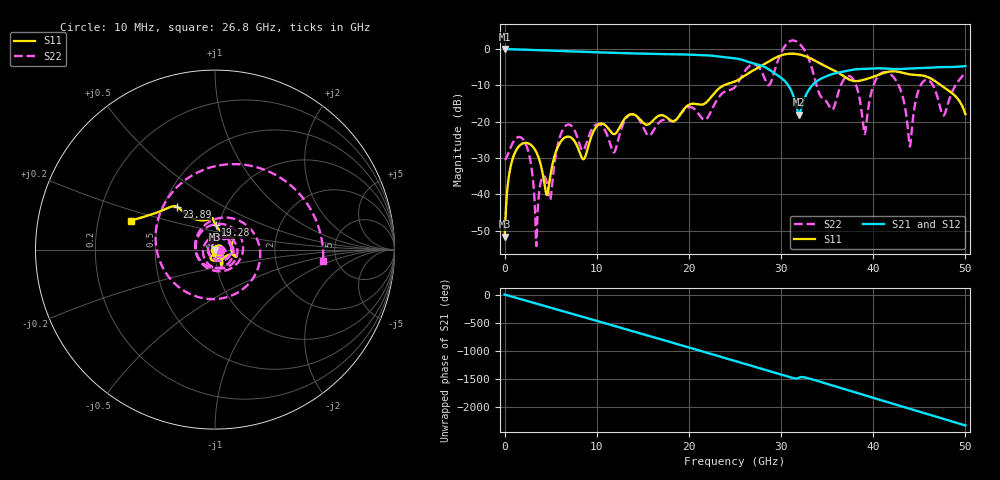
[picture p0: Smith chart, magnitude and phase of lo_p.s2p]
!Keysight Technologies,N5245B,MY57181346,A.12.70.07
!Automatic Fixture Removal (AFR)
!Date: Tuesday, November 06, 2018 3:02:35 PM
!S2P File: Measurements: S11,S21,S12,S22:
# MHz S  RI  R 50
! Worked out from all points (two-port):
!   5000 points, 10 MHz to 50 GHz, reference 50 ohm
!   highest |S21| = 0.00 dB at 10 MHz (marker M1); lowest = -18.0 dB at 31.95 GHz (marker M2)
!   |S21| within 3 dB of the highest: start of sweep to 25.83 GHz
!   lowest |S11| = -51.7 dB at 10 MHz (marker M3), VSWR 1.01, Z = 49.7 + j0.0402 ohm
!   |S11| at or under -10 dB: start of sweep to 23.78 GHz; 47.37 GHz to end of sweep
!   |S22| runs from -54.3 to 2.4 dB; largest |S21 - S12| = 1.5e-15
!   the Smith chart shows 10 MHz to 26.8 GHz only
!   S11 on the Smith chart (normalised r, x): 10 MHz: 0.99, +0.00; 19.28 GHz: 0.97, +0.27; 23.89 GHz: 0.59, +0.31; 26.8 GHz: 0.35, +0.15
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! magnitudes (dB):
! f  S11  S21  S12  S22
! 10 MHz  -51.7  0.0  0.0  -30.5
! 1.69 GHz  -26.5  -0.1  -0.1  -24.3
! 3.47 GHz  -28.5  -0.3  -0.3  -53.4
! 4.6 GHz  -40.2  -0.4  -0.4  -36.8
! 6.44 GHz  -24.6  -0.6  -0.6  -21.7
! 8.35 GHz  -29.7  -0.7  -0.7  -27.6
! 16.68 GHz  -18.4  -1.4  -1.4  -20.5
! 19.28 GHz  -17.2  -1.5  -1.5  -17.4
! 23.89 GHz  -9.9  -2.2  -2.2  -11.7
! 25.01 GHz  -8.9  -2.6  -2.6  -10.4
! 26.8 GHz  -6.1  -3.8  -3.8  -4.4
! 28.7 GHz  -3.4  -5.6  -5.6  -9.9
! 31.95 GHz  -1.5  -18.0  -18.0  1.6
! 33.34 GHz  -2.7  -10.1  -10.1  -5.2
! 35.48 GHz  -5.5  -7.0  -7.0  -16.6
! 37.71 GHz  -8.7  -5.7  -5.7  -7.9
! 39.07 GHz  -8.4  -5.5  -5.5  -23.4
! 41.67 GHz  -6.2  -5.4  -5.4  -6.6
! 43.97 GHz  -7.0  -5.3  -5.3  -26.8
! 45.38 GHz  -7.3  -5.2  -5.2  -9.1
! 47.64 GHz  -10.5  -5.0  -5.0  -18.3
! 50 GHz  -17.9  -4.7  -4.7  -6.5
